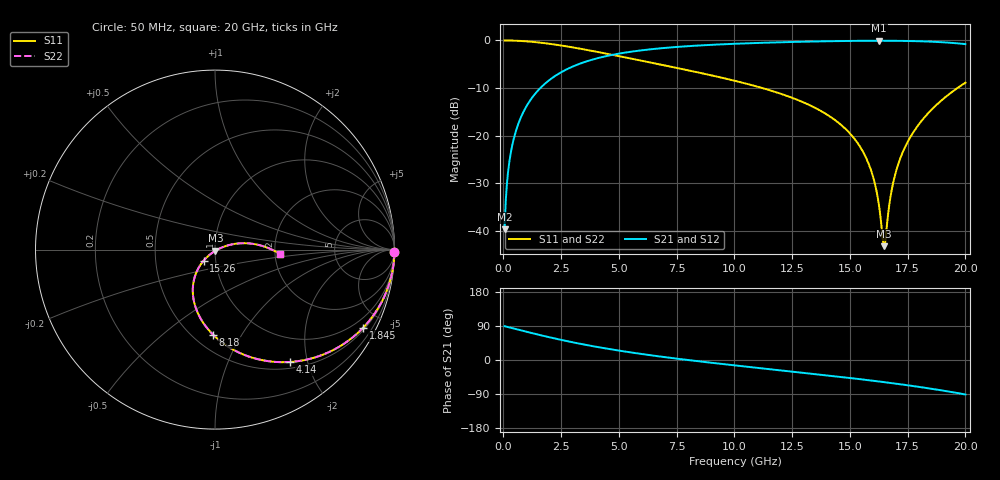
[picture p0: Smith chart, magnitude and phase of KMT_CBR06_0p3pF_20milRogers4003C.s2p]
! Data measured by Modelithics Inc. support@modelithics.com 813-866-6335
! KEMET CBR0603 0.3pF, Pad Width= 0.851mm, Pad Length= 0.64mm, Pad Gap= 0.62mm, 20mil Rogers 4003C substrate Data, January 2022
# hz S ma R 50
! 2 Port Network Data from SP1.SP block
! freq  magS11  angS11  magS21  angS21  magS12  angS12  magS22  angS22
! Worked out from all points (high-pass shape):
!   401 points, 50 MHz to 20 GHz, reference 50 ohm
!   highest |S21| = -0.06 dB at 16.26 GHz (marker M1); lowest = -39.6 dB at 50 MHz (marker M2)
!   |S21| within 3 dB of the highest: 4.676 GHz to end of sweep
!   lowest |S11| = -43.2 dB at 16.46 GHz (marker M3), VSWR 1.01, Z = 50.2 - j0.672 ohm
!   |S11| at or under -10 dB: 11.21 GHz to 19.65 GHz (8.438 GHz wide, 54.7 % of centre)
!   |S22| runs from -43.2 to 0.0 dB; largest |S21 - S12| = 0
!   S11 on the Smith chart (normalised r, x): 50 MHz: open; 1.845 GHz: 0.59, -3.94; 4.14 GHz: 0.59, -1.71; 8.18 GHz: 0.62, -0.76; 15.26 GHz: 0.87, -0.11; 20 GHz: 2.12, -0.11
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5e7  0.9999 -0.8  0.01044 89.2  0.01044 89.2  0.9999 -0.8
2.495e8  0.9986 -3.9  0.05202 86.1  0.05202 86.1  0.9986 -3.9
5.4875e8  0.9935 -8.6  0.1138 81.4  0.1138 81.4  0.9935 -8.6
1.0475e9  0.9768 -16.2  0.2137 73.8  0.2137 73.8  0.9768 -16.2
1.8455e9  0.9326 -27.9  0.3599 62.0  0.3599 62.0  0.9326 -27.9
3.391625e9  0.8136 -48.0  0.5799 41.9  0.5799 41.9  0.8136 -48.0
4.13975e9  0.7522 -56.3  0.6572 33.5  0.6572 33.5  0.7522 -56.3
6.73325e9  0.5625 -80.2  0.8243 9.6  0.8243 9.6  0.5625 -80.2
8.179625e9  0.4754 -91.2  0.877 -1.5  0.877 -1.5  0.4754 -91.2
1.0025e10  0.3767 -103.8  0.923 -14.2  0.923 -14.2  0.3767 -103.8
1.336662e10  0.2032 -125.1  0.9746 -36.2  0.9746 -36.2  0.2032 -125.1
1.446388e10  0.1394 -131.7  0.985 -43.7  0.985 -43.7  0.1394 -131.7
1.526188e10  0.08852 -135.8  0.9902 -49.3  0.9902 -49.3  0.08852 -135.8
1.591025e10  0.04369 -136.2  0.9926 -54.0  0.9926 -54.0  0.04369 -136.2
1.625938e10  0.01852 -126.6  0.9929 -56.7  0.9929 -56.7  0.01852 -126.6
1.645888e10  0.006921 -75.3  0.9928 -58.2  0.9928 -58.2  0.006921 -75.3
1.655862e10  0.008903 -18.3  0.9927 -59.0  0.9927 -59.0  0.008903 -18.3
1.670825e10  0.01909 8.4  0.9923 -60.2  0.9923 -60.2  0.01909 8.4
1.705738e10  0.04731 17.9  0.9908 -63.0  0.9908 -63.0  0.04731 17.9
1.770575e10  0.1049 16.8  0.9852 -68.5  0.9852 -68.5  0.1049 16.8
1.870325e10  0.2057 9.3  0.9667 -77.6  0.9667 -77.6  0.2057 9.3
2e10  0.3604 -3.7  0.9152 -91.0  0.9152 -91.0  0.3604 -3.7
